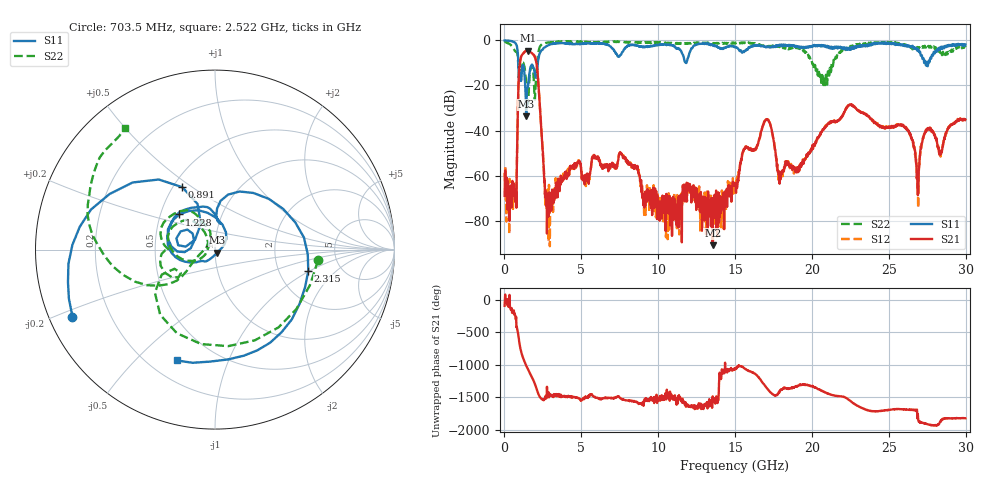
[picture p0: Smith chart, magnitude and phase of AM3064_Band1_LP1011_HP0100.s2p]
# Hz S DB R 50.0
!freq dBS11 angS11 dBS21 angS21 dBS12 angS12 dBS22 angS22
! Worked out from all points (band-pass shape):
!   1600 points, 10 MHz to 29.98 GHz, reference 50 ohm
!   highest |S21| = -4.52 dB at 1.51 GHz (marker M1); lowest = -90.8 dB at 13.54 GHz (marker M2)
!   |S21| within 3 dB of the highest: 1.074 GHz to 1.988 GHz (914.1 MHz wide, 59.7 % of centre)
!   lowest |S11| = -33.6 dB at 1.416 GHz (marker M3), VSWR 1.04, Z = 51.2 - j1.73 ohm
!   |S11| at or under -10 dB: 902.1 MHz to 2.166 GHz (1.264 GHz wide, 82.4 % of centre); 27.39455 GHz to 27.45872 GHz (64.17 MHz wide, 0.234 % of centre); 27.49002 GHz to 27.56234 GHz (72.32 MHz wide, 0.263 % of centre)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
!   |S22| runs from -28.2 to -0.4 dB; largest |S21 - S12| = 0.0071
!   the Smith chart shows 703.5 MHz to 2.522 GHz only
!   S11 on the Smith chart (normalised r, x): 703.5 MHz: 0.07, -0.22; 891 MHz: 0.56, +0.46; 1.228 GHz: 0.63, +0.27; 2.315 GHz: 2.93, -0.97; 2.522 GHz: 0.31, -0.67
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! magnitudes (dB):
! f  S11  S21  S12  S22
! 10 MHz  -0.1  -69.0  -58.8  -0.4
! 703.5 MHz  -1.1  -66.2  -67.4  -4.8
! 891 MHz  -8.1  -25.0  -24.9  -9.7
! 1.228 GHz  -11.1  -5.8  -5.7  -10.0
! 1.416 GHz  -33.6  -4.6  -4.6  -18.6
! 1.51 GHz  -20.8  -4.5  -4.5  -25.9
! 2.315 GHz  -5.5  -30.7  -30.6  -2.7
! 2.522 GHz  -3.7  -53.4  -52.4  -1.5
! 2.803 GHz  -2.3  -68.9  -66.1  -1.0
! 5.015 GHz  -1.4  -59.1  -57.2  -0.8
! 7.601 GHz  -6.1  -50.5  -50.2  -0.7
! 10 GHz  -2.0  -73.5  -72.7  -1.0
! 13.54 GHz  -2.3  -90.8  -77.4  -1.3
! 15 GHz  -2.9  -63.1  -65.8  -1.4
! 17.03 GHz  -3.1  -34.9  -34.9  -2.8
! 17.91 GHz  -2.0  -62.0  -61.7  -2.7
! 19.99 GHz  -2.9  -48.2  -48.0  -9.4
! 22.48 GHz  -3.7  -28.6  -28.5  -2.7
! 25 GHz  -1.0  -38.3  -38.4  -1.1
! 26.89 GHz  -4.1  -68.7  -62.5  -3.5
! 27.45 GHz  -10.2  -39.9  -39.5  -2.5
! 29.98 GHz  -1.8  -35.1  -35.3  -3.0
